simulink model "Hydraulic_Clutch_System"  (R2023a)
settings: Solver=VariableStepAuto  StartTime=0.0  StopTime=10.0  RelTol=1e-3
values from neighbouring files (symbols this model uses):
  A_p = 1    [Hydraulic_Clutch_System_EQN.m]    (also in Hydraulic_Clutch_System_SLX_m.m)
undefined symbols (not defined in the file or in its folder): iGm
libraries: fl_lib x9, nesl_utility x1

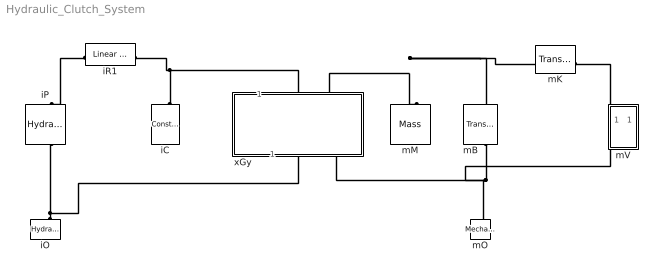
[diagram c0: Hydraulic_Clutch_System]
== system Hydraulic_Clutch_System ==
  iC : fl_lib/Hydraulic/Hydraulic Elements/Constant Volume Hydraulic Chamber  ch_sp=foundation.enum.chamberGeometry.volume  wall_type=foundation.enum.chamber_spec.rigid  ch_volume=1e-4 m^3  d_in=1e-2 m  length=1 m  pr_r_coef=1.2e-12 m/Pa  time_const=0.01 s  k_sh=1.4  pressure_specify=off  pressure_priority=High  pressure=0 Pa  pressure_nominal_specify=off  pressure_nominal_unit=Pa  pressure_nominal_value=1  diameter_incr_specify=off  diameter_incr_priority=High  diameter_incr=0 m  diameter_incr_nominal_specify=off  diameter_incr_nominal_unit=m  diameter_incr_nominal_value=1  flow_rate_specify=off  flow_rate_priority=None  flow_rate=1e-3 m^3/s  flow_rate_nominal_specify=off  flow_rate_nominal_unit=m^3/s  flow_rate_nominal_value=1
  iO : fl_lib/Hydraulic/Hydraulic Elements/Hydraulic Reference
  iP : fl_lib/Hydraulic/Hydraulic Sources/Hydraulic Constant Pressure Source  commanded_pressure=10e5 Pa
  iR1 : fl_lib/Hydraulic/Hydraulic Elements/Linear Hydraulic Resistance  resistance=10e9 Pa*s/m^3  q_specify=off  q_priority=None  q=1e-3 m^3/s  q_nominal_specify=off  q_nominal_unit=m^3/s  q_nominal_value=1  p_specify=off  p_priority=None  p=0 Pa  p_nominal_specify=off  p_nominal_unit=Pa  p_nominal_value=1
  mB : fl_lib/Mechanical/Translational Elements/Translational Damper  D=100 N*s/m  v_specify=off  v_priority=None  v=0 m/s  v_nominal_specify=off  v_nominal_unit=m/s  v_nominal_value=1  f_specify=off  f_priority=None  f=0 N  f_nominal_specify=off  f_nominal_unit=N  f_nominal_value=1
  mK : fl_lib/Mechanical/Translational Elements/Translational Spring  spr_rate=1000 N/m  v_specify=off  v_priority=None  v=0 m/s  v_nominal_specify=off  v_nominal_unit=m/s  v_nominal_value=1  f_specify=off  f_priority=None  f=0 N  f_nominal_specify=off  f_nominal_unit=N  f_nominal_value=1  x_specify=off  x_priority=High  x=0 m  x_nominal_specify=off  x_nominal_unit=m  x_nominal_value=1
  mM : fl_lib/Mechanical/Translational Elements/Mass  mass=1 kg  num_ports=foundation.enum.numPorts2.one  v_specify=off  v_priority=High  v=0 m/s  v_nominal_specify=off  v_nominal_unit=m/s  v_nominal_value=1  f_specify=off  f_priority=None  f=0 N  f_nominal_specify=off  f_nominal_unit=N  f_nominal_value=1
  mO : fl_lib/Mechanical/Translational Elements/Mechanical Translational Reference
  mV : Subsystem  mask{mV='Va'}
      mask prompts: mV "Output variable"
  xGy : Subsystem  mask{Gyrator_type=iGm, G_type=F2=K*E1, xGy=A_p}
      mask prompts: Gyrator_type "Type of Gytator"; G_type "Type of relation"; xGy "Name of parameter K"
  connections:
  iR1/LConn1 -- iP/LConn1
  iC/LConn1 -- xGy/LConn1 -- iR1/RConn1
  iO/LConn1 -- iP/RConn1 -- xGy/RConn1
  xGy/LConn2 -- mB/LConn1 -- mK/LConn1 -- mM/LConn1
  mB/RConn1 -- mO/LConn1 -- mV/RConn1 -- xGy/RConn2
  mK/RConn1 -- mV/LConn1

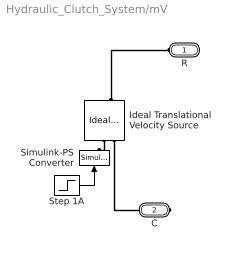
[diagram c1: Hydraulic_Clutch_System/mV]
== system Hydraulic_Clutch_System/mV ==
  Ideal Translational Velocity Source : fl_lib/Mechanical/Mechanical Sources/Ideal Translational Velocity Source
  Simulink-PS Converter : nesl_utility/Simulink-PS Converter  PhysicalDomain=network_engine_domain  SubClassName=ps_input  LeftPortType=input  RightPortType=output  PseudoPeriodic=off  Frequencies=[]  NoiseDistribution=none  NoiseParameters=[]  Unit=1  AffineConversion=off  FilteringAndDerivatives=zero  SimscapeFilterOrder=1  InputFilterTimeConstant=.001  UdotUserProvided=0
  Step 1A : Step  After=100  SampleTime=0
  R : PMIOPort  Side=Left
  C : PMIOPort  Port=2  Side=Right
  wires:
  Step 1A/1 -> Simulink-PS Converter/1
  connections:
  Ideal Translational Velocity Source/RConn1 -- Simulink-PS Converter/RConn1
  Ideal Translational Velocity Source/LConn1 -- R/RConn1
  Ideal Translational Velocity Source/RConn2 -- C/RConn1

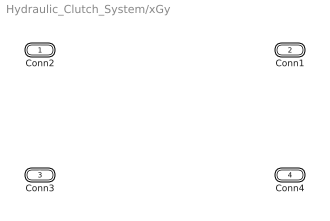
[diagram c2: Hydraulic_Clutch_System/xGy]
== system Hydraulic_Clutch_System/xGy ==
  Conn2 : PMIOPort  Side=Left
  Conn1 : PMIOPort  Port=2  Side=Left
  Conn3 : PMIOPort  Port=3  Side=Right
  Conn4 : PMIOPort  Port=4  Side=Right
